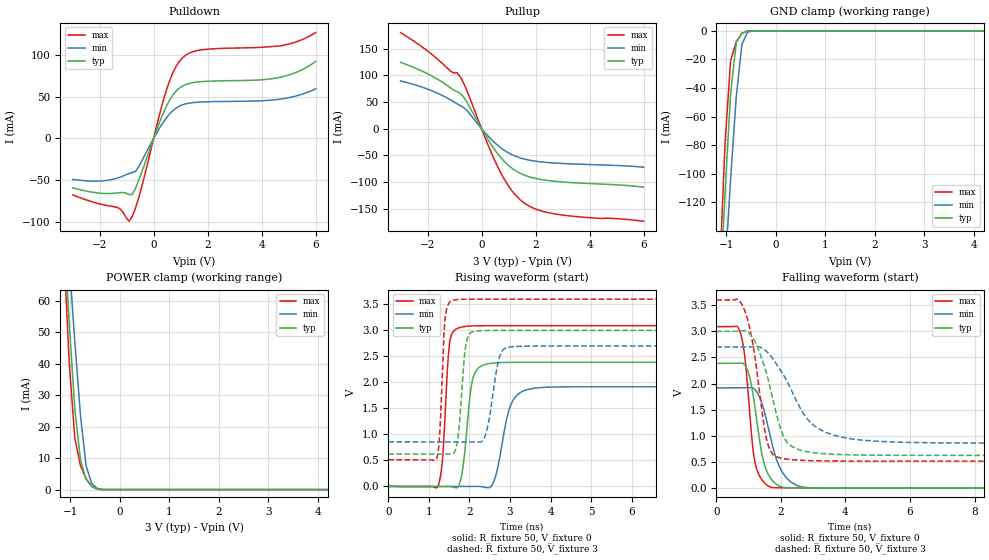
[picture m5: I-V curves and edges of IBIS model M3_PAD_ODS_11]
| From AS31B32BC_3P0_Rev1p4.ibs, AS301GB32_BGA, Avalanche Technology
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[Model] M3_PAD_ODS_11
Model_type I/O
Enable   Active-High
Vinl  =  0.8
Vinh  =  2.2
Vmeas =  1.5
Cref  =  30e-12
| Capacitance  typ   min   max
C_comp   1.536816e-12   1.424706e-12   1.652746e-12
| Variables   typ   min   max
[GND Clamp Reference]   0   0   0
[POWER Clamp Reference]   3   2.7   3.6
[Pulldown Reference]   0   0   0
[Pullup Reference]   3   2.7   3.6
[Temperature Range]   25   125   -40
[Voltage Range]   3   2.7   3.6
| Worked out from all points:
|   slope of the pulldown table from 0 to 0.45 V, typ, clamps not added: 12.2 ohm
|   slope of the pullup table from 0 to 0.45 V, typ, clamps not added: 12.3 ohm
|   GND clamp passes 1 mA (typ) near -0.63 V on its own axis
|   POWER clamp passes 1 mA (typ) near -0.57 V on its own axis
|   falling waveform, R_fixture 50, V_fixture 0: 20-80 % time 370ps typ, 517ps min, 271ps max; typ from 2.39 V to 0 V
|   falling waveform, R_fixture 50, V_fixture 3: 20-80 % time 631ps typ, 1.06ns min, 432ps max; typ from 3 V to 0.623 V
|   rising waveform, R_fixture 50, V_fixture 0: 20-80 % time 184ps typ, 299ps min, 130ps max; typ from 0 V to 2.39 V
|   rising waveform, R_fixture 50, V_fixture 3: 20-80 % time 139ps typ, 221ps min, 101ps max; typ from 0.623 V to 3 V
[GND Clamp]
| Voltage   I(typ)   I(min)   I(max)
-3V       -1.712A    -1.49A     -2.05A
-1.138V   -196mA     -238.3mA   -175.4mA
-1.024V   -114.1mA   -169mA     -78.8mA
-910.3mV  -43.65mA   -103.4mA   -20.77mA
-796.6mV  -8.267mA   -46.07mA   -7.668mA
-682.8mV  -1.833mA   -9.55mA    -1.767mA
-569mV    -178.4uA   -969.7uA   -71.94uA
-455.2mV  -3.831uA   -72.48uA   -403.8nA
6V        0A         0A         0A
[POWER Clamp]
| Voltage   I(typ)   I(min)   I(max)
-3V       673.8mA    591mA      808.5mA
-1.138V   84.79mA    99.96mA    78.44mA
-1.024V   53.08mA    72.89mA    40.56mA
-910.3mV  25.62mA    46.98mA    16.4mA
-796.6mV  9.531mA    23.75mA    7.632mA
-682.8mV  3.235mA    7.564mA    3.468mA
-569mV    995.3uA    1.941mA    1.029mA
-455.2mV  154.7uA    390.4uA    112.5uA
-227.6mV  35.58nA    2.313uA    2.593nA
6V        0A         0A         0A
[Pulldown]
| Voltage   I(typ)   I(min)   I(max)
-3V       -59.47mA   -49.3mA    -67.99mA
-1.252V   -65.23mA   -46.75mA   -84.53mA
-910.3mV  -67.62mA   -42.31mA   -99.67mA
-796.6mV  -67.5mA    -41.16mA   -93.98mA
-569mV    -51.9mA    -35.1mA    -73.18mA
206.9mV   18.25mA    11.68mA    27.22mA
517.2mV   41.4mA     26.44mA    62.3mA
827.6mV   56.6mA     36.23mA    86.17mA
1.241V    65.21mA    41.79mA    100.9mA
1.966V    68.46mA    43.86mA    107mA
4.49V     72.13mA    46.26mA    110.5mA
6V        92.39mA    59.42mA    127mA
[Pullup]
| Voltage   I(typ)   I(min)   I(max)
-3V       124.2mA    89.58mA    180mA
-1.821V   98.19mA    70.66mA    138.4mA
-1.138V   76.16mA    53.74mA    107.4mA
-796.6mV  66.5mA     43.37mA    97.71mA
-569mV    51.88mA    35.59mA    74.49mA
103.4mV   -9.007mA   -6.076mA   -13.35mA
620.7mV   -48.21mA   -31.99mA   -73.47mA
1.034V    -70.25mA   -46.17mA   -109.9mA
1.552V    -86.01mA   -56.24mA   -137.9mA
2.069V    -93.69mA   -61.15mA   -151.5mA
2.793V    -98.65mA   -64.34mA   -160mA
6V        -109.3mA   -71.93mA   -173.1mA
[Ramp]
dV/dt_r   1.432/0.184458n  1.14988/0.298556n  1.85402/0.129888n
dV/dt_f   1.42647/0.630613n  1.10595/1.05796n  1.85298/0.431635n
R_load = 50
[Falling Waveform]
R_fixture = 50
V_fixture = 0
V_fixture_min = 0
V_fixture_max = 0
| Time   V(typ)   V(min)   V(max)
0s        2.387V     1.916V     3.09V
739.8ps   2.391V     1.917V     2.983V
889.6ps   2.351V     1.917V     2.482V
1.054ns   2.074V     1.922V     1.296V
1.189ns   1.589V     1.889V     516.5mV
1.432ns   591.9mV    1.586V     138.6mV
1.721ns   154.5mV    861.2mV    8.015mV
2.125ns   5.714mV    228.9mV    1.346mV
2.749ns   1.114mV    8.253mV    703.6uV
21.88ns   568.2nV    538.1nV    -524.3nV
[Falling Waveform]
R_fixture = 50
V_fixture = 3
V_fixture_min = 2.7
V_fixture_max = 3.6
| Time   V(typ)   V(min)   V(max)
0s        3V         2.7V       3.6V
663ps     3.001V     2.701V     3.616V
867.2ps   3.017V     2.701V     3.421V
1.163ns   2.843V     2.713V     2.652V
1.556ns   2.196V     2.615V     933.4mV
2.018ns   1.09V      2.229V     568mV
2.308ns   807mV      1.897V     541.5mV
2.965ns   678mV      1.227V     520.5mV
4.374ns   630.7mV    924.2mV    512.6mV
21.88ns   622.5mV    856.7mV    511.7mV
[Rising Waveform]
R_fixture = 50
V_fixture = 0
V_fixture_min = 0
V_fixture_max = 0
| Time   V(typ)   V(min)   V(max)
0s        2.964nV    37.59nV    -5.714nV
1.225ns   777.8uV    541.9uV    8.251mV
1.333ns   846.3uV    589.5uV    501.5mV
1.512ns   473.7uV    669uV      2.769V
1.856ns   468.6mV    821.1uV    3.07V
2.093ns   2.102V     925.9uV    3.085V
2.511ns   2.365V     -12.99mV   3.09V
3.031ns   2.385V     1.587V     3.09V
3.633ns   2.387V     1.891V     3.09V
21.88ns   2.387V     1.916V     3.09V
[Rising Waveform]
R_fixture = 50
V_fixture = 3
V_fixture_min = 2.7
V_fixture_max = 3.6
| Time   V(typ)   V(min)   V(max)
0s        622.5mV    856.8mV    511.7mV
1.196ns   622.3mV    856.4mV    548.6mV
1.271ns   622.3mV    856.3mV    1.073V
1.398ns   622.3mV    856.3mV    3.212V
1.6ns     633.3mV    856.2mV    3.582V
1.72ns    951.5mV    856.2mV    3.592V
1.914ns   2.733V     856.1mV    3.598V
2.142ns   2.982V     856.1mV    3.599V
3.008ns   2.999V     2.68V      3.599V
21.88ns   3V         2.7V       3.6V
